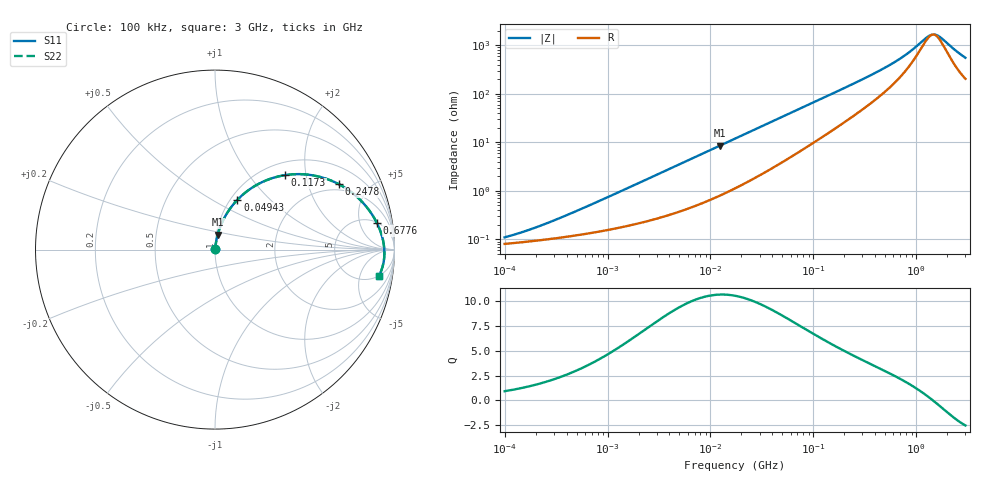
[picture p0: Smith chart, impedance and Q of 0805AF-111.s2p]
# MHz  S  MA  R  50
!Freq  MagS11  AngS11  MagS21  AngS21  MagS12  AngS12  MagS22  AngS22
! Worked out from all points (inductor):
!   801 points, 100 kHz to 3 GHz, reference 50 ohm
!   read as one part in series: L = 116 nH near 501.3 kHz
!   highest Q = 10.7 at 12.28 MHz (marker M1), where L = 109 nH
!   self-resonance near 1.453 GHz
!   S11 on the Smith chart (normalised r, x): 100 kHz: 1.00, +0.00; 49.43 MHz: 1.08, +0.66; 117.3 MHz: 1.24, +1.53; 247.8 MHz: 1.71, +3.18; 677.6 MHz: 5, +9; 3 GHz: 5, -10
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0.1  0.001097 42.9  0.9992 -0.0  0.9992 -0.0  0.001097 42.9
0.2085689  0.001807 58.5  0.9991 -0.1  0.9991 -0.1  0.001807 58.5
0.5630108  0.004277 72.7  0.9987 -0.2  0.9987 -0.2  0.004277 72.7
3.129194  0.02217 81.7  0.997 -1.3  0.997 -1.3  0.02217 81.7
12.27792  0.08377 79.9  0.9887 -4.8  0.9887 -4.8  0.08377 79.9
17.39195  0.117 77.9  0.9821 -6.7  0.9821 -6.7  0.117 77.9
31.07331  0.2017 72.5  0.9589 -11.6  0.9589 -11.6  0.2017 72.5
49.43322  0.3043 65.8  0.918 -17.6  0.918 -17.6  0.3043 65.8
69.12602  0.3991 59.3  0.867 -23.3  0.867 -23.3  0.3991 59.3
96.66387  0.5064 51.6  0.7918 -30.1  0.7918 -30.1  0.5064 51.6
117.2944  0.5701 46.7  0.7371 -34.3  0.7371 -34.3  0.5701 46.7
168.3068  0.6823 37.4  0.6173 -42.1  0.6173 -42.1  0.6823 37.4
247.8151  0.7803 27.8  0.4786 -49.6  0.4786 -49.6  0.7803 27.8
364.8832  0.8498 19.6  0.3481 -55.0  0.3481 -55.0  0.8498 19.6
544.228  0.8963 12.7  0.233 -57.4  0.233 -57.4  0.8963 12.7
677.6347  0.9137 9.4  0.1792 -56.6  0.1792 -56.6  0.9137 9.4
888.4111  0.9291 5.8  0.1212 -51.4  0.1212 -51.4  0.9291 5.8
1274.789  0.9412 1.5  0.06414 -22.9  0.06414 -22.9  0.9412 1.5
1469.088  0.9435 -0.1  0.05659 2.2  0.05659 2.2  0.9435 -0.1
1693.002  0.9441 -1.8  0.06358 27.6  0.06358 27.6  0.9441 -1.8
2429.304  0.9373 -6.2  0.1219 56.0  0.1219 56.0  0.9373 -6.2
3000  0.9259 -9.0  0.1678 59.4  0.1678 59.4  0.9259 -9.0
